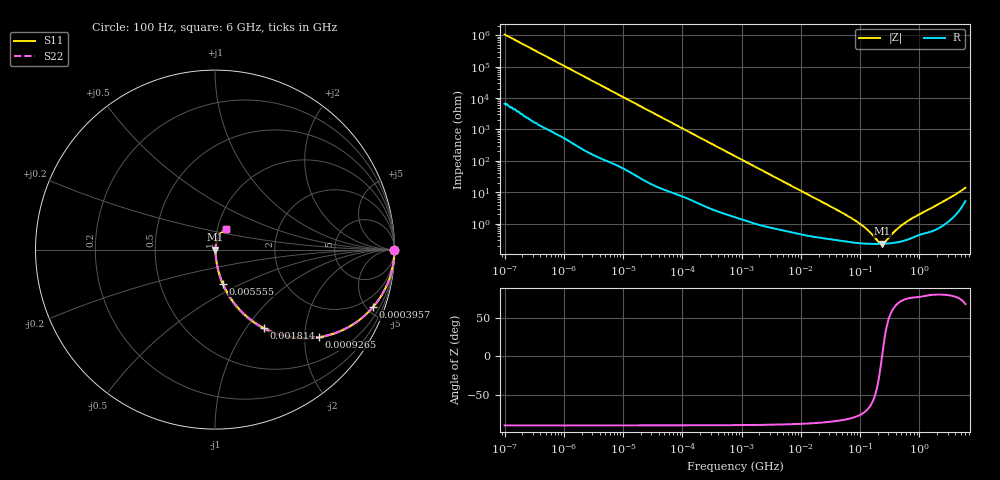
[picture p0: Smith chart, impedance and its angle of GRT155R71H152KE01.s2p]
!Murata Part Number: GRT155R71H152KE01
!These Parameters are Measured in Series Mode Connection
!Data Generated on Jun 19, 2026
!  o--ll--o
!Port1  Port2
!  o------o
!Operation Temp=25[degC], DC Bias Voltage=0[V]
!Freq. Start=100[Hz] Stop=6[GHz] 401[Steps]
# Hz S RI R 50
!Freq.(Hz) S11(Real) S11(Imag) S21(Real) S21(Imag) S12(Real) S12(Imag) S22(Real) S22(Imag)
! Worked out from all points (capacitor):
!   401 points, 100 Hz to 6 GHz, reference 50 ohm
!   read as one part in series: C = 1.5 nF near 109 Hz
!   lowest |Z| = 229 mohm at 238.8 MHz (marker M1)
!   series resonance near 234.7 MHz, so ESL is about 310 pH
!   S11 on the Smith chart (normalised r, x): 100 Hz: open; 395.7 kHz: 1.05, -5.50; 926.5 kHz: 1.03, -2.36; 1.814 MHz: 1.02, -1.21; 5.555 MHz: 1.01, -0.40; 6 GHz: 1.11, +0.26
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100  1 -9.44e-05  6e-07 9.44e-05  6e-07 9.44e-05  1 -9.44e-05
120  1 -0.000113  7e-07 0.000113  7e-07 0.000113  1 -0.000113
2008  1 -0.00188  1.2e-05 0.00188  1.2e-05 0.00188  1 -0.00188
40335  0.9984 -0.0373  0.00159 0.0373  0.00159 0.0373  0.9984 -0.0373
141303  0.9824 -0.1279  0.0176 0.1279  0.0176 0.1279  0.9824 -0.1279
395726  0.8811 -0.3192  0.1189 0.3192  0.1189 0.3192  0.8811 -0.3192
774597  0.6637 -0.4668  0.3363 0.4668  0.3363 0.4668  0.6637 -0.4668
926525  0.5812 -0.4874  0.4188 0.4874  0.4188 0.4874  0.5812 -0.4874
1813585  0.2715 -0.4369  0.7285 0.4369  0.7285 0.4369  0.2715 -0.4369
2967816  0.1261 -0.322  0.8739 0.322  0.8739 0.322  0.1261 -0.322
5554849  0.0434 -0.1898  0.9566 0.1898  0.9566 0.1898  0.0434 -0.1898
1.555665e7  0.00896 -0.071  0.991 0.071  0.991 0.071  0.00896 -0.071
8.527865e7  0.00257 -0.0118  0.9974 0.0118  0.9974 0.0118  0.00257 -0.0118
1.334425e8  0.00232 -0.00593  0.9977 0.00593  0.9977 0.00593  0.00232 -0.00593
2.088084e8  0.00226 -0.00117  0.9977 0.00117  0.9977 0.00117  0.00226 -0.00117
2.388273e8  0.00227 0.000176  0.9977 -0.000176  0.9977 -0.000176  0.00227 0.000176
2.61201e8  0.00229 0.00107  0.9977 -0.00107  0.9977 -0.00107  0.00229 0.00107
3.124326e8  0.00236 0.0029  0.9976 -0.0029  0.9976 -0.0029  0.00236 0.0029
4.470121e8  0.00263 0.00688  0.9974 -0.00688  0.9974 -0.00688  0.00263 0.00688
6.688484e8  0.00336 0.0123  0.9966 -0.0123  0.9966 -0.0123  0.00336 0.0123
3.065283e9  0.0148 0.0592  0.9852 -0.0592  0.9852 -0.0592  0.0148 0.0592
6e9  0.0639 0.1143  0.9361 -0.1143  0.9361 -0.1143  0.0639 0.1143
